TYPE ConfigHighTempChiller :
STRUCT
	LiftServoPosition1:SVLREAL;
	LiftServoPosition2:SVLREAL;
	LiftServoPosition3:SVLREAL;
	LiftServoPosition4:SVLREAL;
	LiftServoPosition5:SVLREAL;
	
	OriginSearchHighSpeed:SVLREAL;
	OriginSearchLowSpeed:SVLREAL;
	
	AbsMoveSpeed:SVLREAL;
	MaxMoveSpeed:SVLREAL;
	
	SoftDownLimit:SVLREAL;
	SoftUpLimit:SVLREAL;
END_STRUCT
END_TYPE
